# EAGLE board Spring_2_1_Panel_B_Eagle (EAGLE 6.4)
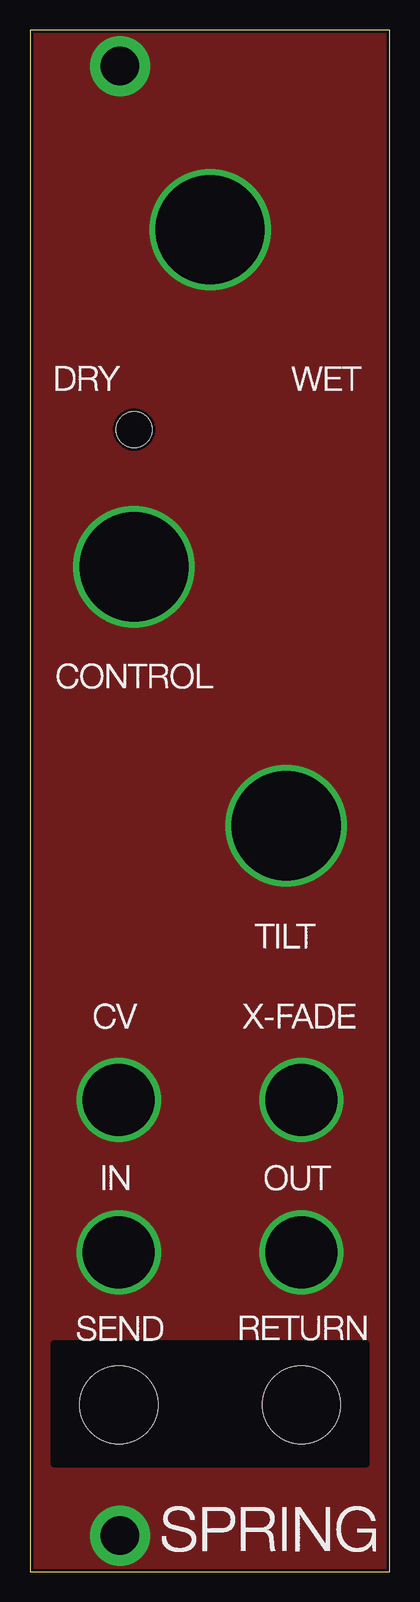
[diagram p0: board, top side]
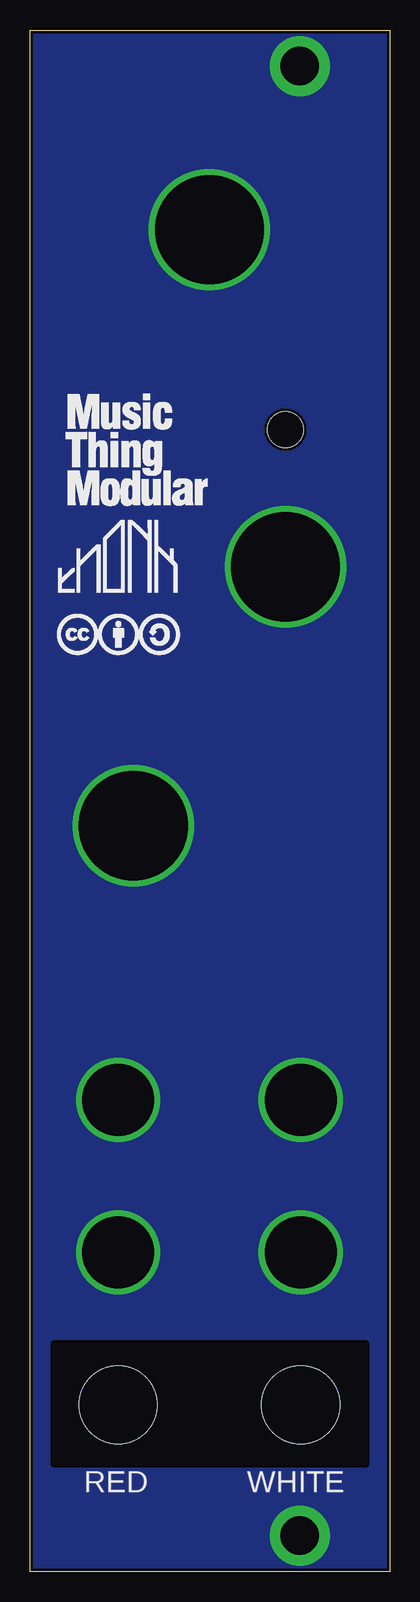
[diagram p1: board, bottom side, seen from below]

Size 30 x 128.5 mm. Coordinates in mm from the lower left corner, seen from the top.
Outline: 0,0 30,0 30,128.5 0,128.5 0,0
Copper layers (1*2*15*16): Top 0.035mm / dielectric 0.2mm / Route2 0.0175mm / dielectric 1.1mm / Route15 0.0175mm / dielectric 0.2mm / Bottom 0.035mm
Design rules "SeeedStudio_DRU_no_angle_20130527": minimum track width 6mil, minimum drill 12mil, track to track 6mil, track to pad 6mil, pad to pad 6mil, via to via 6mil, smd to smd 0mil, copper to edge 10mil, drill to drill 10mil, minimum pad ring 6mil, minimum via ring 6mil, stop-mask expansion 2mil, vias tented up to drill 25mil, thermal gap 10mil
Holes 3 mm at 8.68,95.18
Holes 6.5 mm at 7.41,13.9 22.65,13.9
tRestrict: area 2,9 to 28,19
bRestrict: area 2,9 to 28,19

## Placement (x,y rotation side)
U$1  [MTM_1CM_KEEPOUT]  17.98,78.68 0 top
U$2  [MTM_1CM]  27.1,88.37 0 bottom
U$3  [THONK_1CM_SCREENPRINT]  27.66,81.6 0 bottom
U$4  [CC_1CM_SCREENPRINT]  27.74,76.42 0 bottom

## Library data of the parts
U$1-U$4 = TW_logos

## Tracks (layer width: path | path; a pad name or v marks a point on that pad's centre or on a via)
GND  (via drill 3.2 pad 5, 6, 9.1)
  other vias: 7.5,3 7.5,125.5 22.65,39.3 7.41,39.3 22.65,26.6 7.41,26.6 21.38,62.16 8.68,83.75 15.03,111.85
  pour Bottom: -2.5,132 34.5,132 35.5,-5.5 -2.5,-4
  pour Top: -2.5,130.5 36.5,130.5 36.5,128.5 35,128.5 35,-2.5 -10.5,-2.5 -10.5,1 -4,1 -4,129.5

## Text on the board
bPlace: WHITE | RED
